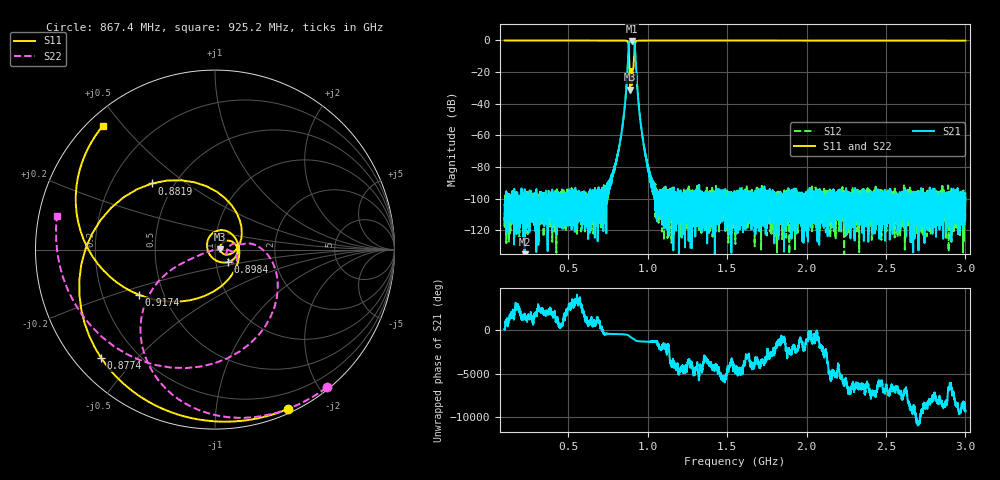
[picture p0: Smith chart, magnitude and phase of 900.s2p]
# Hz S DB R 50
! Planar, S50180, 20087770, 20.1.2/1
! Date: 23.06.2021 14:39:54
! Data: Format (Calibration Info)
! Freq	S11:dB/Ang(F2)	S21:dB/Ang(F2)	S12:dB/Ang(F2)	S22:dB/Ang(F2)
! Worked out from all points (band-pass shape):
!   8991 points, 100 MHz to 3 GHz, reference 50 ohm
!   highest |S21| = -0.54 dB at 901.3 MHz (marker M1); lowest = -146.3 dB at 225.5 MHz (marker M2)
!   |S21| within 3 dB of the highest: 881.3 MHz to 919.1 MHz (37.75 MHz wide, 4.19 % of centre)
!   lowest |S11| = -31.1 dB at 889.7 MHz (marker M3), VSWR 1.06, Z = 52.9 + j0.152 ohm
!   |S11| at or under -10 dB: 883.6 MHz to 915.1 MHz (31.52 MHz wide, 3.51 % of centre)
!   |S22| runs from -45.3 to 0.0 dB; largest |S21 - S12| = 0.0017
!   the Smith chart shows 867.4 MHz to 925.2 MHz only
!   S11 on the Smith chart (normalised r, x): 867.4 MHz: 0.04, -1.56; 877.4 MHz: 0.08, -0.40; 881.9 MHz: 0.38, +0.38; 898.4 MHz: 1.14, -0.16; 917.4 MHz: 0.36, -0.24; 925.2 MHz: 0.04, +0.44
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1e8  0.02 154.2  -103.74 147.0  -116.20 -41.0  0.01 150.4
2.254839e8  -0.01 123.4  -146.32 -170.4  -97.90 -84.9  -0.00 116.7
5.835484e8  -0.01 52.8  -100.65 82.7  -101.75 -53.4  0.01 43.6
7.919355e8  -0.01 9.2  -81.51 -82.6  -81.14 -87.7  0.01 3.7
8.364516e8  -0.02 -13.3  -58.03 -105.8  -58.09 -105.3  -0.01 -14.8
8.551613e8  -0.07 -34.8  -42.78 -125.0  -42.77 -125.1  -0.03 -30.6
8.674194e8  -0.20 -65.3  -28.27 -151.4  -28.26 -151.6  -0.10 -51.0
8.774194e8  -1.15 -136.4  -10.70 150.1  -10.70 150.0  -0.82 -93.1
8.819355e8  -5.87 133.5  -2.80 81.7  -2.79 81.6  -5.09 -137.4
8.896774e8  -31.11 3.0  -0.61 -36.9  -0.61 -36.8  -45.26 -1.2
8.983871e8  -20.02 -44.3  -0.57 -134.9  -0.58 -134.8  -19.01 -37.8
9.012903e8  -27.31 -122.9  -0.54 -166.0  -0.54 -166.0  -23.31 -20.5
9.174194e8  -6.12 -149.5  -2.24 -6.2  -2.24 -6.2  -6.27 -50.3
9.251613e8  -0.62 132.1  -13.12 -115.8  -13.12 -115.8  -0.91 168.0
9.429032e8  -0.12 74.9  -39.48 167.0  -39.46 166.8  -0.12 73.9
9.603226e8  -0.06 54.8  -55.62 143.3  -55.60 143.4  -0.04 48.7
9.909677e8  -0.01 37.3  -74.67 123.7  -74.32 125.5  -0.00 29.2
1.066774e9  -0.01 17.2  -104.80 33.7  -109.68 30.9  0.04 9.2
1.55e9  -0.01 -35.8  -120.21 -115.8  -111.46 122.0  0.03 -40.4
2.033548e9  -0.04 -73.8  -106.85 109.1  -109.53 109.7  -0.01 -75.3
2.516774e9  -0.07 -108.9  -103.94 133.6  -103.45 67.4  -0.05 -107.5
3e9  -0.11 -145.3  -101.63 124.4  -94.91 -39.1  -0.09 -140.7
